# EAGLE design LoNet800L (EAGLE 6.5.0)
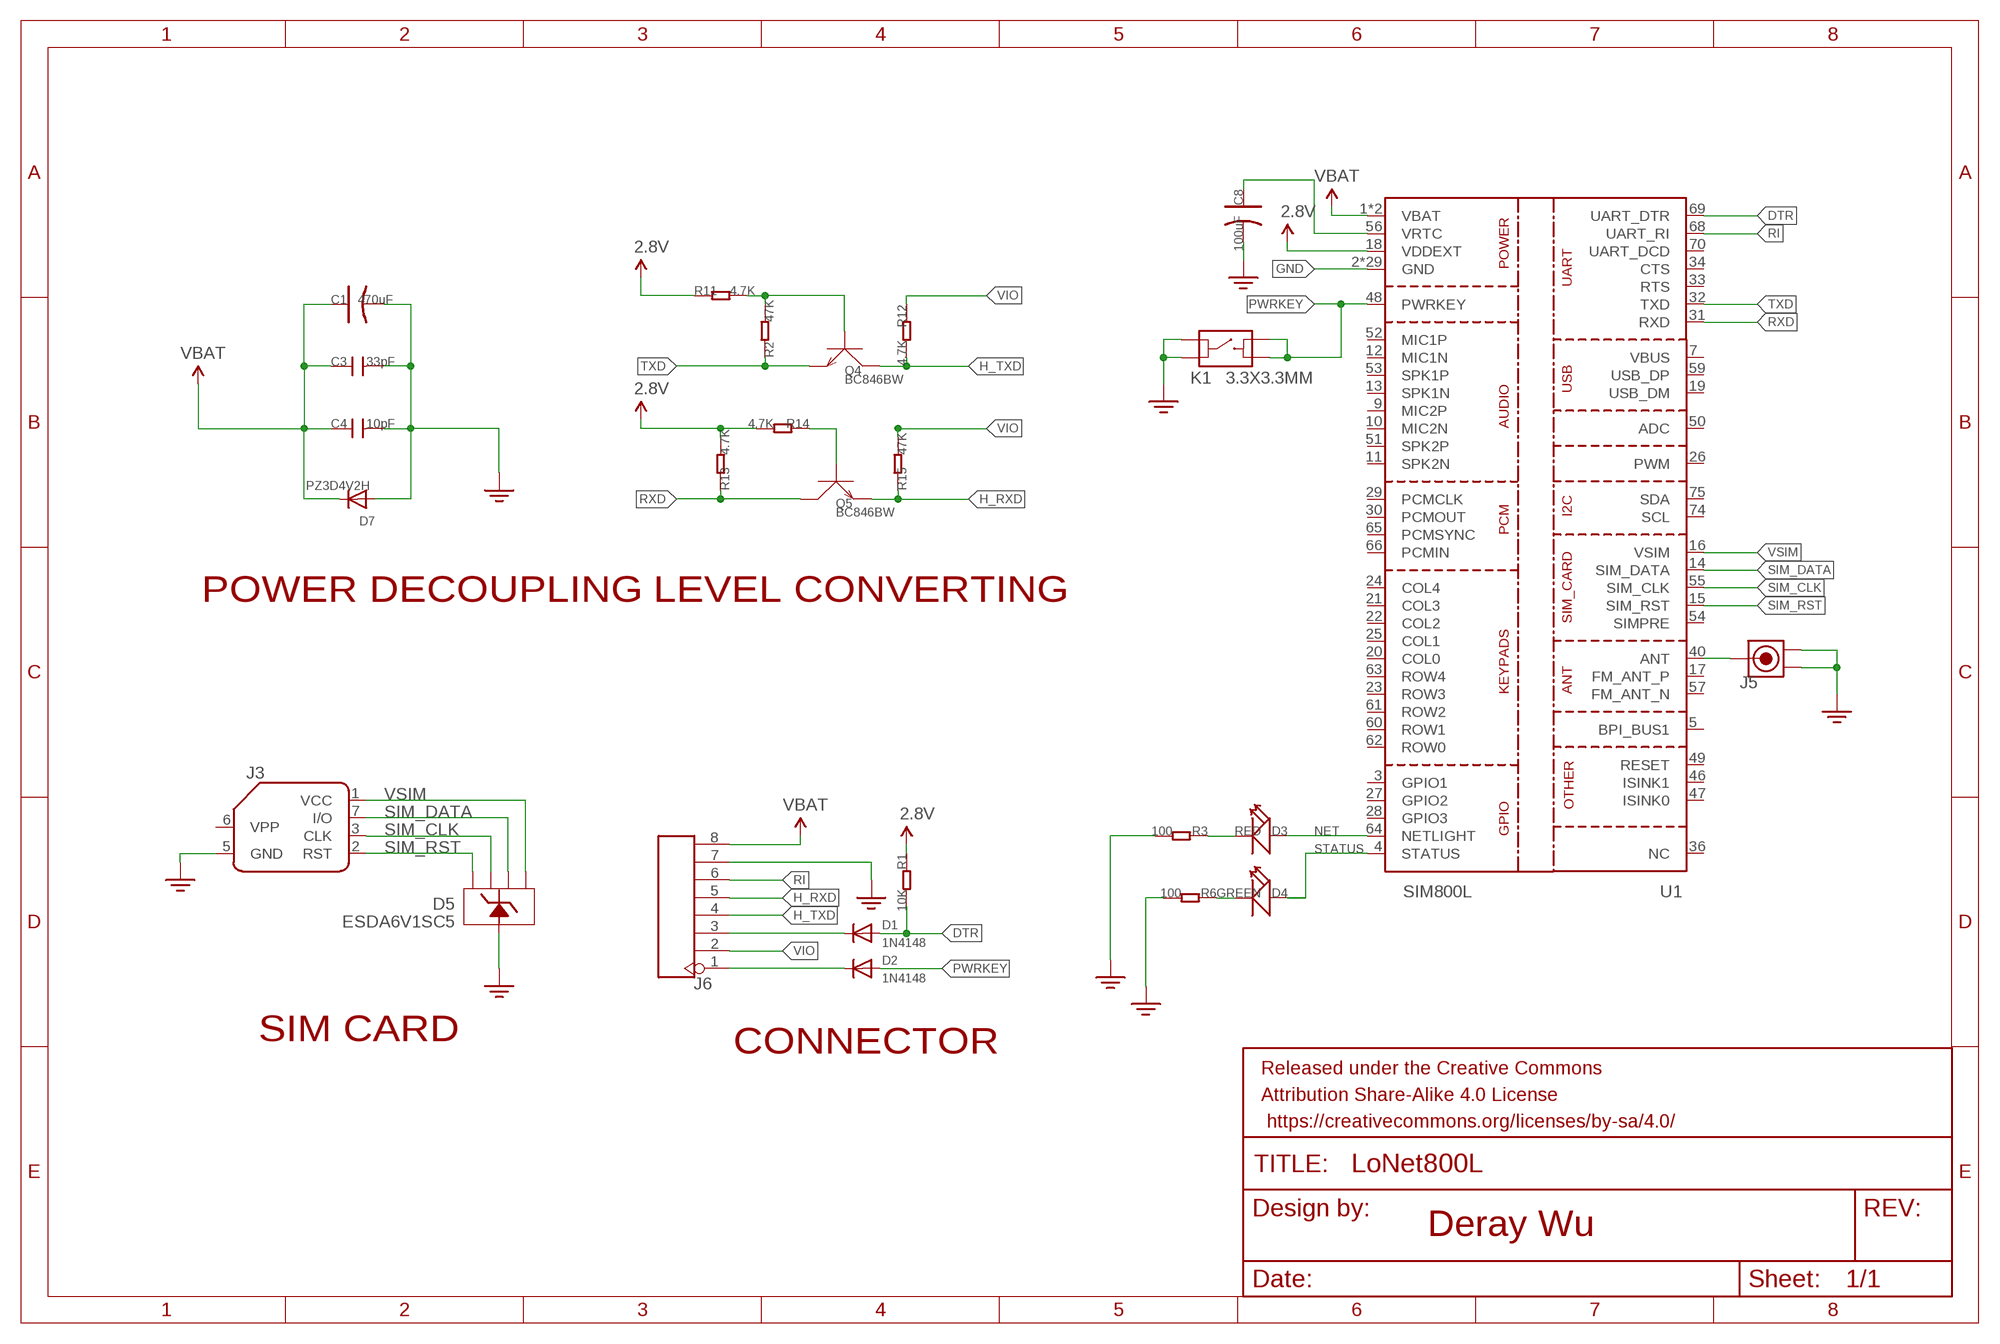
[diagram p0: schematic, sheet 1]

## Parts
C1  470uF  CAP-AVX-D  [AVX-D]
C3  33pF  C-0603  [C0603]
C4  10pF  C-0603  [C0603]
C8  100uF  CAP-AVX-A  [AVX-A]
D1  1N4148  DIODESOD-323F  [SOD-323F]
D2  1N4148  DIODESOD-323F  [SOD-323F]
D3  RED  LED-0603  [0603]
D4  GREEN  LED-0603  [0603]
D5  ESDA6V1SC5  D-ESD-ESDA6V1SC5-SOT23-5L  [SOT23-5L]
D7  PZ3D4V2H  DIODESOD-323F  [SOD-323F]
J3  SIMHOLDERSIM  [SIMHOLDER]
J5  ANTENNA-U-FL'3PAD-TYPE'  [3P-U-FL]
J6  HEADER-8P-2.54  [8P-2.54]
K1  3.3X3.3MM  BUTTON-4P-3.3X3.3  [4P-SMD-3.4X3.4X1.3H]
Q4  BC846BW  TRANSISTOR-NPN-SOT323  [SOT323]
Q5  BC846BW  TRANSISTOR-NPN-SOT323  [SOT323]
R1  10K  R-0603  [0603]
R2  47K  R-0603  [0603]
R3  100  R-0603  [0603]
R6  100  R-0603  [0603]
R11  4.7K  R-0603  [0603]
R12  4.7K  R-0603  [0603]
R13  4.7K  R-0603  [0603]
R14  4.7K  R-0603  [0603]
R15  47K  R-0603  [0603]
U1  SIM800L  [88P-17.8X15.8X2.4]

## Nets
2.8V: R1.1 R11.1 R13.2 R14.2 U1.18(VDDEXT)
ANT: J5.D U1.40(ANT)
DTR: D1.A R1.2 U1.69(UART_DTR)
GND: C1.- C3.2 C4.2 C8.- D5.2 D7.A J3.5(GND) J5.GND1 J5.GND2 J6.7 K1.A0 K1.A1 R3.2 R6.2 U1.2(GND) U1.6(GND) U1.8(GND) U1.35(GND) U1.37(GND) U1.38(GND) U1.39(GND) U1.41(GND) U1.43(GND) U1.44(GND) U1.45(GND) U1.58(GND) U1.67(GND) U1.71(GND) U1.72(GND) U1.73(GND) U1.76(GND) U1.77(GND) U1.78(GND) U1.79(GND) U1.80(GND) U1.81(GND) U1.82(GND) U1.83(GND) U1.84(GND) U1.85(GND) U1.86(GND) U1.87(GND) U1.88(GND)
H_DTR: D1.C J6.3
H_RXD: J6.5 Q5.2(E) R15.1
H_TXD: J6.4 Q4.3(C) R12.2
N$1: C8.+ U1.56(VRTC)
N$4: D3.- R3.1
N$6: Q4.1(B) R2.2 R11.2
N$8: D4.- R6.1
N$9: Q5.1(B) R14.1
NET: D3.+ U1.64(NETLIGHT)
PWR: D2.C J6.1
PWRKEY: D2.A K1.B0 K1.B1 U1.48(PWRKEY)
RI: J6.6 U1.68(UART_RI)
RXD: Q5.3(C) R13.1 U1.31(RXD)
SIM_CLK: D5.5 J3.3(CLK) U1.55(SIM_CLK)
SIM_DATA: D5.3 J3.7(I/O) U1.14(SIM_DATA)
SIM_RST: D5.4 J3.2(RST) U1.15(SIM_RST)
STATUS: D4.+ U1.4(STATUS)
TXD: Q4.2(E) R2.1 U1.32(TXD)
VBAT: C1.+ C3.1 C4.1 D7.C J6.8 U1.1(VBAT) U1.42(VBAT)
VIO: J6.2 R12.1 R15.2
VSIM: D5.1 J3.1(VCC) U1.16(VSIM)
Unconnected: J3.6(VPP) U1.3(GPIO1) U1.5(BPI_BUS1) U1.7(VBUS) U1.9(MIC2P) U1.10(MIC2N) U1.11(SPK2N) U1.12(MIC1N) U1.13(SPK1N) U1.17(FM_ANT_P) U1.19(USB_DM) U1.20(COL0) U1.21(COL3) U1.22(COL2) U1.23(ROW3) U1.24(COL4) U1.25(COL1) U1.26(PWM) U1.27(GPIO2) U1.28(GPIO3) U1.29(PCMCLK) U1.30(PCMOUT) U1.33(RTS) U1.34(CTS) U1.36(NC) U1.46(ISINK1) U1.47(ISINK0) U1.49(RESET) U1.50(ADC) U1.51(SPK2P) U1.52(MIC1P) U1.53(SPK1P) U1.54(SIMPRE) U1.57(FM_ANT_N) U1.59(USB_DP) U1.60(ROW1) U1.61(ROW2) U1.62(ROW0) U1.63(ROW4) U1.65(PCMSYNC) U1.66(PCMIN) U1.70(UART_DCD) U1.74(SCL) U1.75(SDA)

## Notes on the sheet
- POWER DECOUPLING | LEVEL CONVERTING
- SIM CARD
- CONNECTOR
- Deray Wu

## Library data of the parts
C1 = Common:CAP*
C3 C4 = Capacitors:C*
C8 = Capacitors:CAP*
D1 D2 D7 = Semiconductors:DIODE: Diode
D3 D4 = LEDs:LED*
D5 = Semiconductors:D-ESD-ESDA6V1SC5: Quad Transil array for ESD protection STMicroelectronics http://www.st.com/internet/com/TECHNICAL_RESOURCES/TECHNICAL_LITERATURE/DATASHEET/CD00002055.pdf
J3 = SparkFun-Connectors:SIMHOLDER: SIM Socket Socket for SIM cellular cards. Schematic element and footprint production proven. Spark Fun Electronics SKU : PRT-00548; PROD_ID: CONN-08536
J5 = Connector:ANTENNA-U-FL
J6 = Connector:HEADER-8P
K1 = Buttons:BUTTON-4P
Q4 Q5 = Semiconductors:TRANSISTOR-NPN*: NPN audion
R1-R3 R6 R11-R15 = Resistors:R*
U1 = SIMCOM:SIM800L

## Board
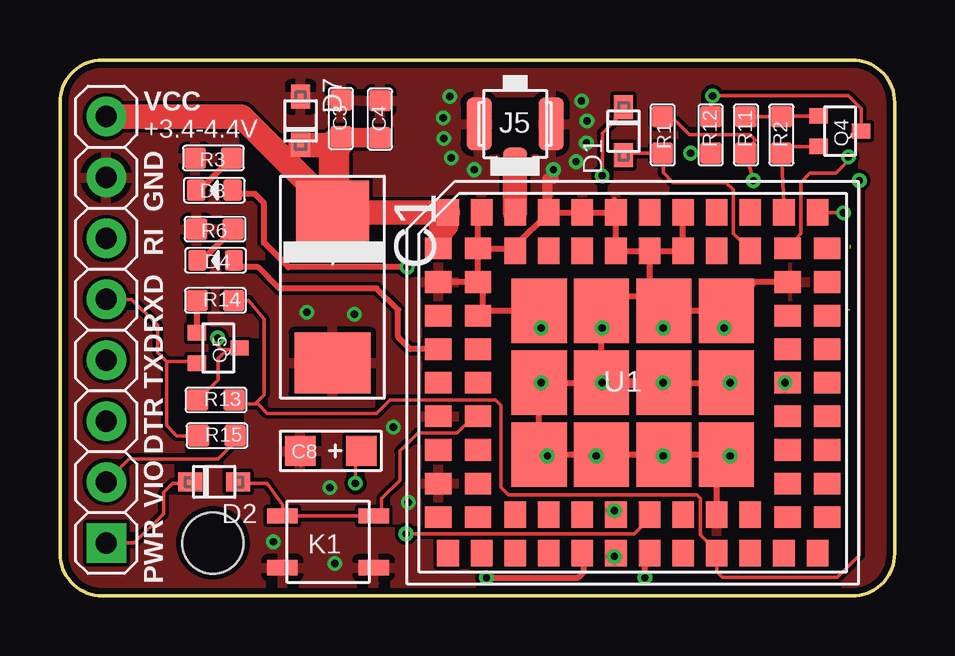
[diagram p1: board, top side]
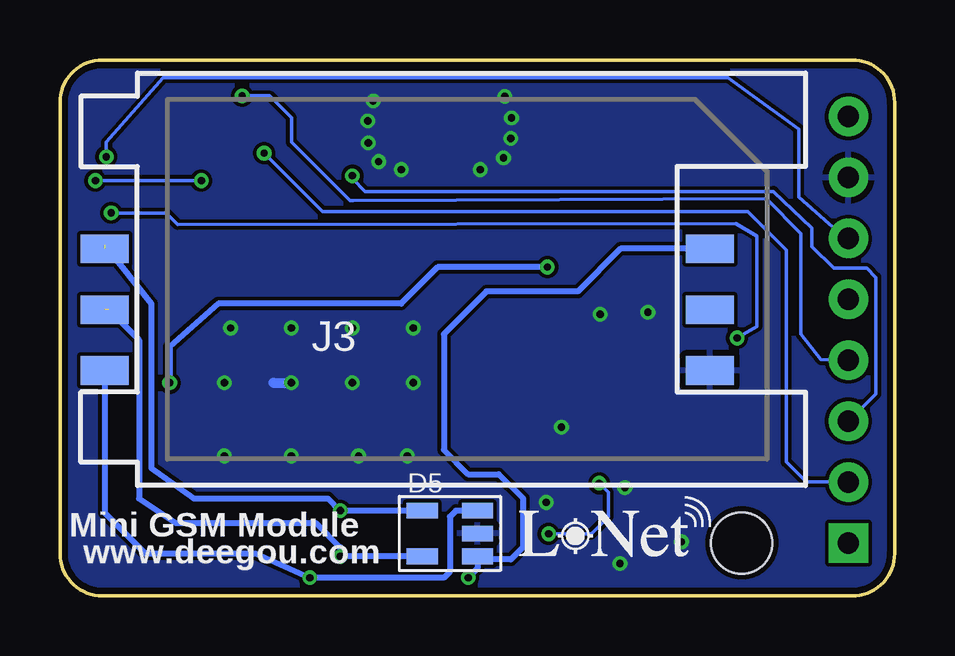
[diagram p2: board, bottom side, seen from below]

Size 34.8 x 22.35 mm. Coordinates in mm from the lower left corner, seen from the top.
Outline: 34.8,20.57 arc90 33.02,22.35 1.78,22.35 arc90 0,20.57 0,1.78 arc90 1.78,0 33.02,0 arc90 34.8,1.78 34.8,20.57
Copper layers (1*2*15*16): Top 0.035mm / dielectric 0.2mm / Route2 0.0175mm / dielectric 1.1mm / Route15 0.0175mm / dielectric 0.2mm / Bottom 0.035mm
Design rules "DRU": minimum track width 6mil, minimum drill 12mil, track to track 6mil, track to pad 6mil, pad to pad 6mil, via to via 6mil, smd to smd 0mil, copper to edge 10mil, drill to drill 10mil, minimum pad ring 6mil, minimum via ring 6mil, stop-mask expansion 2mil, vias tented up to drill 25mil, thermal gap 10mil
Holes 2.54 mm at 6.38,2.21
tRestrict: area 16.8,3 to 30.2,16.5

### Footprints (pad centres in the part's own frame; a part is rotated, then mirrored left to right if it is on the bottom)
AVX-D = smd 2.54 x 3.048: + -3.175,0 | smd 2.54 x 3.175: - 3.175,0
C0603 = smd 0.889 x 0.889: 1 -0.762,0; 2 0.762,0
AVX-A = smd 1.27 x 1.27: + -1.27,0; - 1.27,0
SOD-323F = smd 1 x 0.8: A -1,0; C 1,0
0603 = smd 0.762 x 0.889: + -0.762,0; - 0.762,0
SOT23-5L = smd 0.65 x 1.3: 1 0,1.15; 2 0.95,1.15; 3 1.9,1.15; 4 1.9,-1.15; 5 0,-1.15
SIMHOLDER = smd 2 x 1.2: 1 -12.61,-3.81; 2 -12.61,-1.27; 3 -12.61,1.27; 5 12.61,-3.81; 6 12.61,-1.27; 7 12.61,1.27
3P-U-FL = smd 1.05 x 1: D -1.524,0 | smd 2.2 x 1.05: GND1 0,1.5; GND2 0,-1.5
8P-2.54 = drill 0.889 pad 1.651 square: 1 0,8.89 | drill 0.889 pad 1.651: 2 0,6.35; 3 0,3.81; 4 0,1.27; 5 0,-1.27; 6 0,-3.81; 7 0,-6.35; 8 0,-8.89
4P-SMD-3.4X3.4X1.3H = smd 1.27 x 0.635: A0 -1.905,1.079; A1 1.905,1.079; B0 -1.905,-1.079; B1 1.905,-1.079
SOT323 = smd 0.635 x 0.762: 1 -0.635,-0.889; 2 0.635,-0.889; 3 0,0.889
0603' = smd 0.889 x 0.889: 1 -0.762,0; 2 0.762,0
88P-17.8X15.8X2.4 = smd 1.1 x 0.9: 1 -8.1,5.6; 2 -8.1,4.2; 3 -8.1,2.8; 4 -8.1,1.4; 5 -8.1,0; 6 -8.1,-1.4; 7 -8.1,-2.8; 8 -8.1,-4.2; 9 -8.1,-5.6; 22 8.1,-5.6; 23 8.1,-4.2; 24 8.1,-2.8; 25 8.1,-1.4; 26 8.1,0; 27 8.1,1.4; 28 8.1,2.8; 29 8.1,4.2; 30 8.1,5.6; 43 -6.45,5.6; 44 -6.45,4.2; 45 -6.45,2.8; 46 -6.45,1.4; 47 -6.45,0; 48 -6.45,-1.4; 49 -6.45,-2.8; 50 -6.45,-4.2; 51 -6.45,-5.6; 60 6.45,-5.6; 61 6.45,-4.2; 62 6.45,-2.8; 63 6.45,-1.4; 64 6.45,0; 65 6.45,1.4; 66 6.45,2.8; 67 6.45,4.2; 68 6.45,5.6 | smd 0.9 x 1.1: 10 -7.7,-7.1; 11 -6.3,-7.1; 12 -4.9,-7.1; 13 -3.5,-7.1; 14 -2.1,-7.1; 15 -0.7,-7.1; 16 0.7,-7.1; 17 2.1,-7.1; 18 3.5,-7.1; 19 4.9,-7.1; 20 6.3,-7.1; 21 7.7,-7.1; 31 7.7,7.1; 32 6.3,7.1; 33 4.9,7.1; 34 3.5,7.1; 35 2.1,7.1; 36 0.7,7.1; 37 -0.7,7.1; 38 -2.1,7.1; 39 -3.5,7.1; 40 -4.9,7.1; 41 -6.3,7.1; 42 -7.7,7.1; 52 -4.9,-5.5; 53 -3.5,-5.5; 54 -2.1,-5.5; 55 -0.7,-5.5; 56 0.7,-5.5; 57 2.1,-5.5; 58 3.5,-5.5; 59 4.9,-5.5; 69 4.9,5.5; 70 3.5,5.5; 71 2.1,5.5; 72 0.7,5.5; 73 -0.7,5.5; 74 -2.1,5.5; 75 -3.5,5.5; 76 -4.9,5.5 | smd 2.3 x 2.7: 77 -3.9,3; 78 -3.9,0; 79 -3.9,-3; 80 -1.3,-3; 81 1.3,-3; 82 3.9,-3; 83 3.9,0; 84 3.9,3; 85 1.3,3; 86 -1.3,3; 87 -1.3,0; 88 1.3,0

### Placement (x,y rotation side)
C1  11.36,12.88 270 top
C3  11.71,19.91 90 top
C4  13.34,19.88 90 top
C8  11.29,6.05 180 top
D1  23.5,19.38 90 top
D2  6.43,4.75 180 top
D3  6.44,16.92 180 top
D4  6.49,14 180 top
D5  18.54,3.56 270 bottom
D7  10.03,19.81 270 top
J3  20.32,13.21 0 bottom
J5  18.97,19.69 90 top
J6  1.93,11.1 180 top
K1  11.18,2.26 180 top
Q4  32.51,19.38 270 top
Q5  6.6,10.34 270 top
R1  10K  [0603']  25.12,19.23 270 top
R2  47K  [0603']  30.07,19.23 90 top
R3  100  [0603']  6.4,18.26 180 top
R6  100  [0603']  6.47,15.3 180 top
R11  4.7K  [0603']  28.6,19.23 90 top
R12  4.7K  [0603']  27.13,19.23 90 top
R13  4.7K  [0603']  6.51,8.17 0 top
R14  4.7K  [0603']  6.48,12.32 0 top
R15  47K  [0603']  6.55,6.69 0 top
U1  23.88,8.89 0 top

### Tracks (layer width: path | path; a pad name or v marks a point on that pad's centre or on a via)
2.8V  (via drill 0.3 pad 0.61)
  Top 0.152: v28.91,17.32 R11.1 28.98,19 28.75,19.23 26.24,19.23 25.63,19.84 R1.1 | v33.32,17.32 33.32,1.7 32.41,0.79 27.61,0.79 27.38,1.02 U1.18 27.38,1.86 26.7,2.54 26.7,4.06 26.54,4.22 18.69,4.22 18.39,4.52 18.39,7.95 18.16,8.18 13.77,8.18 13.21,7.62 8.64,7.62 8.25,8 8.13,8 | 8.13,8 7.35,8 R13.2 | R14.2 7.87,12.32 8.51,11.56 8.51,8.38 8.13,8
  Bottom 0.152: v28.91,17.32 v33.32,17.32
ANT
  Top 0.813: U1.40
  Top 1.016: J5.D U1.40
DTR
  Top 0.152: U1.69 28.78,14.4 28.07,15.11 28.07,16.94 27.76,17.25 25.55,17.25 25.15,17.65 25.15,18.44 R1.2 23.58,18.47 D1.A
GND  (via drill 0.3 pad 0.61)
  Top 0.152: 10.03,5.44 C8.-
  Top 0.254: U1.67 28.98,13.09 U1.84 U1.85 24.58,12.49 | U1.72 24.58,12.49 | U1.72 U1.71 U1.35 | U1.72 U1.73 U1.37 | U1.37 23.18,16.45 23.11,16.51 | 24.58,12.49 23.18,12.49 U1.86 U1.87 U1.78 U1.79 U1.80 U1.81 U1.82 27.38,5.49 U1.58 | U1.77 17.63,11.89 | 17.63,11.89 U1.45 | 17.63,11.89 17.63,12.89 U1.44 | U1.44 U1.2 | U1.44 U1.43 | U1.43 17.43,15.84 U1.41 | U1.43 18.88,14.49 U1.76 18.98,14.59 U1.39 U1.38 U1.37 | U1.88 U1.83
  Top 0.406: U1.39 20.32,15.99 20.32,17.4 20.57,17.4 v20.57,17.78 | U1.87 23.24,8.89 v25.15,8.89 U1.88
  Bottom 0.406: 25.91,8.89 v25.15,8.89
  other vias: 20.32,5.84 22.35,5.84 25.15,5.84 27.94,5.84 27.94,8.89 27.69,11.18 25.15,11.18 22.61,11.18 20.07,11.18 20.07,8.89 22.61,8.89 11.46,1.35 21.95,18.9 21.97,19.81 21.74,20.65 16,19.08 15.98,19.94 16.26,20.83 17.27,17.78 16.31,18.26 21.51,18.11 14.52,3.9 13.89,7.04 8.89,2.26 11.25,4.52 12.27,11.75 10.29,11.84
  pour Top: 35.81,-1.02 -1.27,-1.02 -1.27,23.11 36.07,23.11
  pour Bottom: 35.31,-1.27 -0.51,-1.27 -0.51,23.37 35.31,23.37
H_DTR  (via drill 0.3)
  Top 0.152: 23.82,20.7 D1.C 23.5,20.19 22.61,19.3 v22.61,17.53
  Bottom 0.152: J6.3 0.79,8.43 0.79,13.28 1.17,13.66 2.54,13.66 3.45,14.58 3.45,15.34 5.05,16.87 22.07,16.87 22.61,17.4 v22.61,17.53
H_RXD
  Top 0.152: J6.5 3,12.37 4.06,11.3 4.06,10.16 4.45,9.78 | 5.64,9.52 Q5.2 5.64,9.78 4.45,9.78 | R15.1 4.87,6.69 4.45,7.11 4.45,9.78
H_TXD  (via drill 0.3 pad 0.61)
  Top 0.152: Q4.3 33.4,20.32 32.87,20.85 v27.2,20.85 27.13,20.78 R12.2
  Bottom 0.152: J6.4 3.07,9.85 3.91,10.92 3.91,15.11 5.36,16.56 22.58,16.48 22.71,16.48 25.15,18.92 25.15,19.94 26.06,20.85 v27.2,20.85
N$1  (via drill 0.3)
  Top 0.152: U1.56 24.58,3.24 23.95,2.59 v14.43,2.59 | C8.+ 12.19,5.69 12.32,5.56 v12.32,4.7
  Bottom 0.152: v14.43,2.59 12.65,2.59 11.94,3.3 11.94,4.32 v12.32,4.7
N$4
  Top 0.254: D3.- 5.69,16.79 R3.1
N$6
  Top 0.152: Q4.1 30.2,20.02 R2.2 R11.2
N$8
  Top 0.254: D4.- 5.72,13.8 R6.1
N$9
  Top 0.254: Q5.1 5.71,12.19 R14.1
NET  (via drill 0.3 pad 0.61)
  Top 0.254: v30.23,8.89 29.97,9.24 U1.64 | v14.48,13.72 9.52,13.72 8.51,14.73 8.51,16.38 8.13,16.76 7.23,16.76 D3.+
  Bottom 0.254: v14.48,13.72 19.05,13.72 20.57,12.19 28.19,12.19 30.23,10.41 v30.23,8.89
PWR
  Top 0.152: J6.1 3.1,2.21 4.32,3.43 4.32,4.32 4.7,4.7 5.38,4.7 D2.C
PWRKEY
  Top 0.152: D2.A 7.49,4.7 8.64,4.7 9.27,3.81 K1.B1 K1.B0 13.41,3.42 13.41,4.06 14.17,4.83 14.17,6.04 14.93,6.81 16.56,6.81 17.24,7.49 U1.48
RI  (via drill 0.3 pad 0.61)
  Top 0.152: U1.68 30.89,15.11 30.89,17.25 31.27,17.63 32.33,17.63 32.87,18.16 v32.87,18.31
  Bottom 0.152: J6.6 2.03,14.91 3.99,16.64 3.99,19.46 6.96,21.62 30.51,21.62 32.87,18.92 v32.87,18.31
RXD  (via drill 0.3 pad 0.61)
  Top 0.152: U1.31 32.66,15.99 v32.66,15.98 | v6.57,10.76 6.57,10.44 6.73,10.29 6.99,10.29 | 6.99,10.29 7.43,10.29 Q5.3 | R13.1 5.76,8.17 6.6,9.02 6.6,9.91 6.99,10.29
  Bottom 0.152: v32.66,15.98 30.38,15.98 29.9,15.49 6.63,15.52 5.74,15.01 5.74,11.24 v6.57,10.76
SIM_CLK  (via drill 0.3 pad 0.61)  (1 unrouted)
  Top 0.254: v23.11,3.56 23.11,3.45 U1.55
  Bottom 0.254: 32.93,14.64 30.99,12.19 30.99,5.33 29.21,4.06 23.62,4.06 v23.11,3.56 D5.5
SIM_DATA  (via drill 0.3 pad 0.61)
  Top 0.254: 21.84,1.86 U1.14 | U1.14 21.58,1.79 | v17.78,0.76 21.59,0.76 21.84,1.02 21.84,1.72 U1.14
  Bottom 0.254: J3.7 11.43,14.48 13.21,12.7 17.02,12.7 18.8,10.92 18.8,6.1 17.78,5.08 16.51,5.08 15.49,4.06 15.49,2.03 16,1.52 17.26,1.52 D5.3 17.39,1.15 v17.78,0.76
SIM_RST  (via drill 0.3 pad 0.61)  (1 unrouted)
  Top 0.254: v23.11,1.65 23.11,1.73 U1.15
  Bottom 0.254: 32.77,11.94 31.5,10.67 31.5,4.06 29.97,3.05 24.13,3.05 23.11,2.03 v23.11,1.65 22.47,1.66 D5.4
STATUS
  Top 0.254: U1.4 14.6,10.29 14.1,10.79 14.1,11.94 13.21,12.83 9.14,12.83 8.25,13.72 7.28,13.72 D4.+
TXD
  Top 0.152: U1.32 30.2,15.99 R2.1 30.2,18.75 Q4.2
VBAT
  Top 0.813: U1.1 15.78,15.59 16.07,15.59 16.2,15.46 16.2,15.41 15.95,15.17 15.95,15.09 15.97,15.07 U1.42 | C4.1 11.73,19.12 C3.1 | 10.41,17.14 10.41,16.89 11.43,15.87 | 11.43,18.8 11.43,18.87 C3.1 | C3.1 11.71,18.69 | 11.67,19.19 C3.1
  Top 1.016: J6.8 7.57,19.99 10.41,17.14 10.41,17 C1.+ 11.43,15.99 U1.42 | 11.43,18.8 10.03,18.8 D7.C
  Top 1.27: 11.43,15.87 11.43,18.8
VIO  (via drill 0.3 pad 0.61)
  Top 0.152: v26.29,18.47 R12.1 | R15.2 7.31,6.42 6.6,5.71 2.89,5.71 J6.2
  Bottom 0.152: J6.2 3.68,4.75 4.52,5.59 4.52,14.43 6.12,16.03 23.85,16.03 v26.29,18.47
VSIM  (via drill 0.3 pad 0.61)
  Top 0.254: v24.38,0.76 24.38,1.98 U1.16
  Bottom 0.254: J3.1 32.93,3.47 31.24,1.78 26.67,1.78 v24.38,0.76 18.8,0.76 18.54,1.02 18.54,3.3 18.29,3.56 D5.1

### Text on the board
tPlace: VCC | +3.4-4.4V | GND | RI | RXD | TXD | DTR | VIO | PWR
bPlace: Mini GSM Module | www.deegou.com

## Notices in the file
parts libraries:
Aesthetics: Licensing: Creative Commons ShareAlike 4.0 International - https://creativecommons.org/licenses/by-sa/4.0
Aesthetics: Released under the Creative Commons
Aesthetics: https://creativecommons.org/licenses/by-sa/4.0
